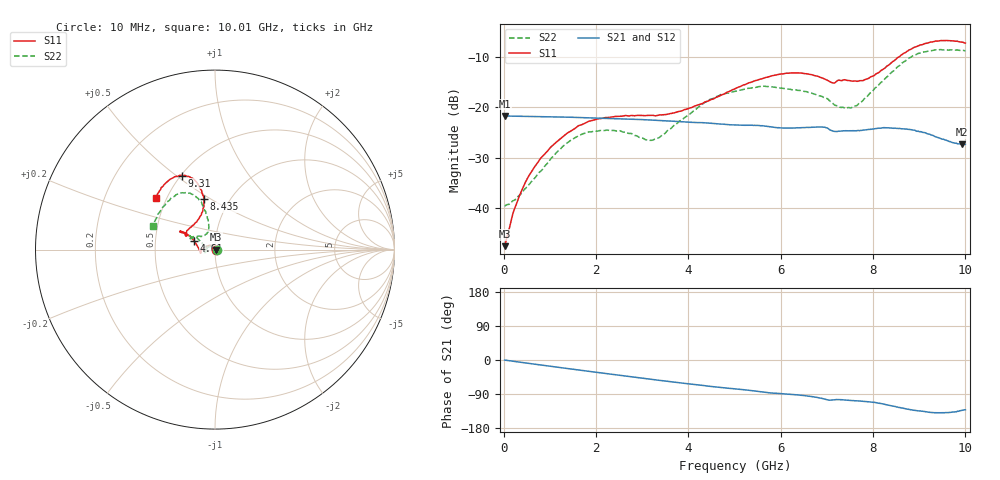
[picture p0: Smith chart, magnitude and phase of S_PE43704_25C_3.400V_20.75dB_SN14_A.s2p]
! Device ID: PE43704
! Dir: z:\PE43704\PE43704_Char_1_20130516\PE43704\AMB\3p400V\20p75dB
! Serial: 14
! Insertion: A
! Impedance: 50 ohm
! Temp: Amb
! VDD: 3.400V
! Attenuation Step: 20.75dB
! IDD: 1.140316e-01mA
#  Hz  S  RI  R  50
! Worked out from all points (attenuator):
!   401 points, 10 MHz to 10.01 GHz, reference 50 ohm
!   highest |S21| = -21.71 dB at 10 MHz (marker M1); lowest = -27.4 dB at 9.935 GHz (marker M2)
!   lowest |S11| = -47.7 dB at 10 MHz (marker M3), VSWR 1.01, Z = 50.4 + j0.0405 ohm
!   |S11| at or under -10 dB: start of sweep to 8.553 GHz
!   |S22| runs from -39.7 to -8.5 dB; largest |S21 - S12| = 0.00093
!   S11 on the Smith chart (normalised r, x): 10 MHz: 1.01, +0.00; 4.61 GHz: 0.79, +0.08; 8.435 GHz: 0.76, +0.46; 9.31 GHz: 0.51, +0.53; 10.01 GHz: 0.44, +0.31
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1e7  0.00412 0.000401  0.0821 -0.000277  0.0821 -0.000214  0.0104 0.000257
2.85e8  0.00119 0.0115  0.0815 -0.0069  0.0814 -0.00685  0.00731 0.0104
6.1e8  -0.0101 0.0212  0.08 -0.0143  0.08 -0.0143  -0.00364 0.0182
1.06e9  -0.0353 0.023  0.0769 -0.0242  0.0769 -0.0241  -0.0272 0.0174
1.685e9  -0.0671 0.00594  0.0703 -0.0366  0.0704 -0.0365  -0.0542 -0.00127
2.235e9  -0.0784 -0.0124  0.0628 -0.0459  0.0629 -0.0458  -0.0576 -0.0149
3.135e9  -0.0814 -0.0174  0.0482 -0.0575  0.0482 -0.0576  -0.0473 -0.000815
3.36e9  -0.0833 -0.0115  0.044 -0.0597  0.044 -0.0595  -0.0492 0.0083
4.61e9  -0.1169 0.0486  0.0218 -0.0652  0.0219 -0.0654  -0.1078 0.0693
5.01e9  -0.1365 0.0699  0.016 -0.065  0.0161 -0.065  -0.1263 0.0708
5.585e9  -0.168 0.0935  0.00665 -0.0653  0.00679 -0.0653  -0.1414 0.0772
5.96e9  -0.1876 0.1017  0.00187 -0.0628  0.00219 -0.0628  -0.1405 0.0694
6.685e9  -0.1886 0.0955  -0.00735 -0.063  -0.00747 -0.0631  -0.1218 0.0652
7.135e9  -0.1563 0.0795  -0.0152 -0.0561  -0.0152 -0.0561  -0.081 0.0737
7.51e9  -0.1392 0.1208  -0.017 -0.0561  -0.017 -0.0559  -0.0488 0.0858
7.86e9  -0.0957 0.1657  -0.0201 -0.0564  -0.0202 -0.0564  -0.0348 0.1212
8.36e9  -0.0613 0.2606  -0.0309 -0.0544  -0.031 -0.0544  -0.0503 0.2055
8.435e9  -0.0627 0.28  -0.0326 -0.0529  -0.0328 -0.0531  -0.0589 0.2212
8.86e9  -0.1021 0.3746  -0.0399 -0.0441  -0.0396 -0.0446  -0.1157 0.3032
9.31e9  -0.183 0.412  -0.0396 -0.0345  -0.0398 -0.0341  -0.2033 0.3099
9.935e9  -0.3168 0.3158  -0.029 -0.0314  -0.0296 -0.0312  -0.3341 0.1603
1.001e10  -0.3281 0.2902  -0.0284 -0.0321  -0.029 -0.0321  -0.3444 0.1306
